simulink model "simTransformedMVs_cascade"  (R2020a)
settings: Solver=ode15s  StartTime=0.0  StopTime=tsim  RelTol=1e-3
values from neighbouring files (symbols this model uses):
  KcTM = 1/kT*tauT/(taucT)    [runTransformedMVsCascade.m]
  KIqM = 1/1.1/(taucq)    (= 18.1818181818)    [runTransformedMVsCascade.m]
  Kparu1 = [0 1]    [runTransformedMVsCascade.m]
  Kparu2 = [1 0]    [runTransformedMVsCascade.m]
  Ku1 = 1/ku1*1/(taucs)    (= 100)    [runTransformedMVsCascade.m]
  Ku2 = 1/ku2*1/(taucs)    (= 100)    [runTransformedMVsCascade.m]
  OL = 1    [SetUpSimulations.m]
  p = [V;A;B; transf]    [runTransformedMVs.m]    (also in runTransformedMVsCascade.m; Main.m = [N, Fc0, rhoc, rhoh,U,A,cpc,cph]; Main_OL.m = [N, Fc0, rhoc, rhoh,U,A,cpc,cph]; runTestCalcBlk.m = [N, Fc0, rhoc, rhoh,U,A,cpc,cph])
  q0 = 10    [SetUpSimulations.m]
  q10 = 5    [SetUpSimulations.m]
  q1f = q10    [runTransformedMVsCascade.m]
  q20 = 5    [SetUpSimulations.m]
  q2f = q20    [runTransformedMVsCascade.m]
  qstep = q0 + 2    (= 12)    [SetUpSimulations.m]
  T0 = 35    [SetUpSimulations.m]    (also in H2P_Turbine_driven.m = param(9); runTD.m = 318; H2P_Boiler_driven.m = param(9); runBD.m = 318)
  T10 = 20    [SetUpSimulations.m]
  T1m = T10    (= 20)    [SetUpSimulations.m]
  T1step = T10 + 10    (= 30)    [SetUpSimulations.m]
  T20 = 50    [SetUpSimulations.m]
  T2m = T20    (= 50)    [SetUpSimulations.m]
  T2step = T20 + 10    (= 60)    [SetUpSimulations.m]
  tauITM = min(-1/A, 4*(taucT))    [runTransformedMVsCascade.m]
  tauTs = 1    [runTransformedMVsCascade.m]
  Tstep = T0 + 10    (= 45)    [SetUpSimulations.m]
  tstep_q = 50    [SetUpSimulations.m]
  tstep_T = 100    [SetUpSimulations.m]
  tstep_T1 = 150    [SetUpSimulations.m]
  tstep_T2 = 200    [SetUpSimulations.m]
  tv1 = 100    [runTransformedMVsCascade.m]
  tv2 = 100    [runTransformedMVsCascade.m]
  vqbias = q0    [runTransformedMVs.m]    (also in runTransformedMVsCascade.m)
  vqbias_step = vqbias    [runTransformedMVs.m]    (also in runTransformedMVsCascade.m)
  vTbias = -A/B*T0    [runTransformedMVs.m]    (also in runTransformedMVsCascade.m)
  vTbias_step = vTbias    [runTransformedMVs.m]    (also in runTransformedMVsCascade.m)
undefined symbols (not defined in the file or in its folder): InputTransf, TempMixDAE

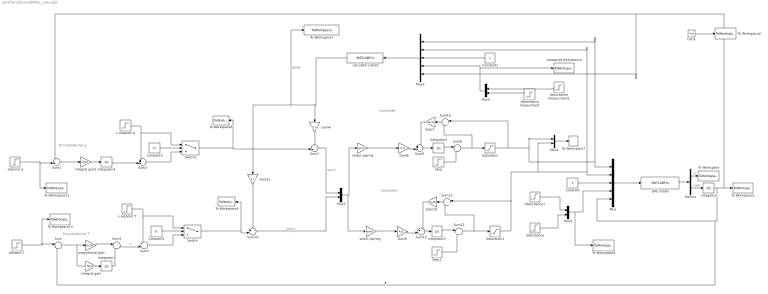
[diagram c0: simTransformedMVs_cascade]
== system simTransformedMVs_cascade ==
  note: I-controller
  note: I-controller
  note: PI-controller for q
  note: PI-controller for T
  " integrator" : Integrator  InitialCondition=T0
  Clock : Clock
  Constant : Constant  Value=p
  Constant1 : Constant  Value=p
  Constant2 : Constant  Value=OL
  Constant3 : Constant  Value=OL
  DAE model : MATLABFcn  MATLABFcn=TempMixDAE(u(1:2), u(3:6),u(7:8),u(9))  OutputDimensions=2
  Demux : Demux  Outputs=2
  Gain10 : Gain  Gain=1/tauTs  Multiplication=Matrix(K*u)
  Gain11 : Gain  Gain=[0 1]  Multiplication=Matrix(K*u)
  Gain4 : Gain  Gain=[1 0]  Multiplication=Matrix(K*u)
  Gain6 : Gain  Gain=Ku1  Multiplication=Matrix(K*u)
  Gain7 : Gain  Gain=1/tauTs  Multiplication=Matrix(K*u)
  Gain9 : Gain  Gain=Ku2  Multiplication=Matrix(K*u)
  Integrator{1..4} (4 alike) : Integrator
  Mux : Mux  Inputs=5
  Mux{1,3..5} (4 alike) : Mux  Inputs=2
  Mux2 : Mux  Inputs=5
  Saturation : Saturate  UpperLimit=inf  LowerLimit=0
  Saturation1 : Saturate  UpperLimit=inf  LowerLimit=0
  Step : Step  Time=tv1  Before=q10  After=q1f  SampleTime=0
  Step1 : Step  Time=tv2  Before=q20  After=q2f  SampleTime=0
  Sum : Sum  Inputs=|+-
  Sum1 : Sum  Inputs=-+|
  Sum10 : Sum  Inputs=|+-
  Sum11 : Sum  Inputs=|+-
  Sum12 : Sum  Inputs=|++
  Sum{2..3,9,13} (4 alike) : Sum  Inputs=++|
  Sum14 : Sum  Inputs=-+|
  Sum4 : Sum  Inputs=|++
  Sum7 : Sum  Inputs=-+|
  Sum8 : Sum  Inputs=|++
  Switch : Switch  Criteria=u2 > Threshold
  Switch1 : Switch  Criteria=u2 > Threshold
  To Workspace : ToWorkspace  VariableName=q  SampleTime=-1
  To Workspace1 : ToWorkspace  VariableName=T  SampleTime=-1
  To Workspace10 : ToWorkspace  VariableName=Tsp  SampleTime=-1
  To Workspace11 : ToWorkspace  VariableName=qsp  SampleTime=-1
  To Workspace2 : ToWorkspace  VariableName=time  SampleTime=-1
  To Workspace3 : ToWorkspace  VariableName=v  SampleTime=-1
  To Workspace4 : ToWorkspace  VariableName=d  SampleTime=-1
  To Workspace5 : ToWorkspace  VariableName=vTs  SampleTime=-1
  To Workspace6 : ToWorkspace  VariableName=vqs  SampleTime=-1
  To Workspace7 : ToWorkspace  VariableName=uplant  SampleTime=-1
  calculate v plant : MATLABFcn  MATLABFcn=InputTransf(u(1:2),u(3:6),u(7:8),u(9))  OutputDimensions=2
  disturbance : Step  Time=tstep_T2  Before=T20  After=T2step  SampleTime=0
  disturbance measurment : Step  Time=tstep_T2  Before=T20  After=T2m  SampleTime=0
  disturbance measurment1 : Step  Time=tstep_T1  Before=T10  After=T1m  SampleTime=0
  disturbance1 : Step  Time=tstep_T1  Before=T10  After=T1step  SampleTime=0
  integral gain : Gain  Gain=KcTM/tauITM  Multiplication=Matrix(K*u)
  integral gain1 : Gain  Gain=KIqM  Multiplication=Matrix(K*u)
  measured disturbance : ToWorkspace  VariableName=dm  SampleTime=-1
  proportional gain : Gain  Gain=KcTM  Multiplication=Matrix(K*u)
  select pairing : Gain  Gain=Kparu1  Multiplication=Matrix(K*u)
  "select pairing   " : Gain  Gain=Kparu2  Multiplication=Matrix(K*u)
  "setpoint T " : Step  Time=tstep_T  Before=T0  After=Tstep  SampleTime=0
  setpoint q : Step  Time=tstep_q  Before=q0  After=qstep  SampleTime=0
  v setpoint T : Step  Time=tstep_T  Before=vTbias  After=vTbias_step  SampleTime=0
  v setpoint q : Step  Time=tstep_q  Before=vqbias  After=vqbias_step  SampleTime=0
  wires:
  DAE model/1 -> Demux/1
  Demux/1 -> To Workspace/1  "q"
  " integrator"/1 -> Sum1/1, Mux2/5, To Workspace1/1, Sum/2, Mux/5  "T"
  Mux/1 -> DAE model/1
  Clock/1 -> To Workspace2/1
  Switch/1 -> To Workspace5/1, Sum14/2
  Demux/2 -> " integrator"/1  "xdot"
  calculate v plant/1 -> Gain11/1, To Workspace3/1, Gain4/1  "vplant"
  Saturation/1 -> Mux2/1, Mux/1, Mux1/1, Sum10/1
  Sum9/1 -> Integrator2/1
  Step/1 -> Sum8/2
  Gain7/1 -> Sum9/1
  Gain6/1 -> Sum9/2
  Gain4/1 -> Sum7/1
  Sum10/1 -> Gain7/1
  Sum8/1 -> Saturation/1, Sum10/2
  Sum12/1 -> Saturation1/1, Sum11/2
  Sum11/1 -> Gain10/1
  Saturation1/1 -> Mux2/2, Mux/2, Mux1/2, Sum11/1
  Gain9/1 -> Sum13/2
  Sum13/1 -> Integrator3/1
  Gain10/1 -> Sum13/1
  Gain11/1 -> Sum14/1
  Constant/1 -> Mux/3
  Mux1/1 -> To Workspace7/1
  Step1/1 -> Sum12/2
  Switch1/1 -> Sum7/2, To Workspace6/1
  Sum7/1 -> Mux3/1  "error1"
  Sum14/1 -> Mux3/2  "error2"
  Mux2/1 -> calculate v plant/1
  Mux4/1 -> measured disturbance/1, Mux2/4
  Constant1/1 -> Mux2/3
  select pairing/1 -> Gain6/1
  Mux3/1 -> "select pairing   "/1, select pairing/1
  "select pairing   "/1 -> Gain9/1
  disturbance measurment/1 -> Mux4/2
  disturbance measurment1/1 -> Mux4/1
  disturbance1/1 -> Mux5/1
  disturbance/1 -> Mux5/2
  Mux5/1 -> To Workspace4/1, Mux/4
  Integrator2/1 -> Sum8/1
  Integrator3/1 -> Sum12/1
  Sum1/1 -> integral gain1/1
  v setpoint q/1 -> Sum2/1, Switch1/1
  Integrator4/1 -> Sum2/2
  Sum2/1 -> Switch1/3
  integral gain1/1 -> Integrator4/1
  Sum/1 -> integral gain/1, proportional gain/1
  Sum4/1 -> Sum3/2  "v"
  Constant3/1 -> Switch1/2
  v setpoint T/1 -> Sum3/1, Switch/1
  Integrator1/1 -> Sum4/2
  proportional gain/1 -> Sum4/1
  setpoint q/1 -> Sum1/2, To Workspace11/1
  Constant2/1 -> Switch/2
  Sum3/1 -> Switch/3
  integral gain/1 -> Integrator1/1
  "setpoint T "/1 -> Sum/1, To Workspace10/1
